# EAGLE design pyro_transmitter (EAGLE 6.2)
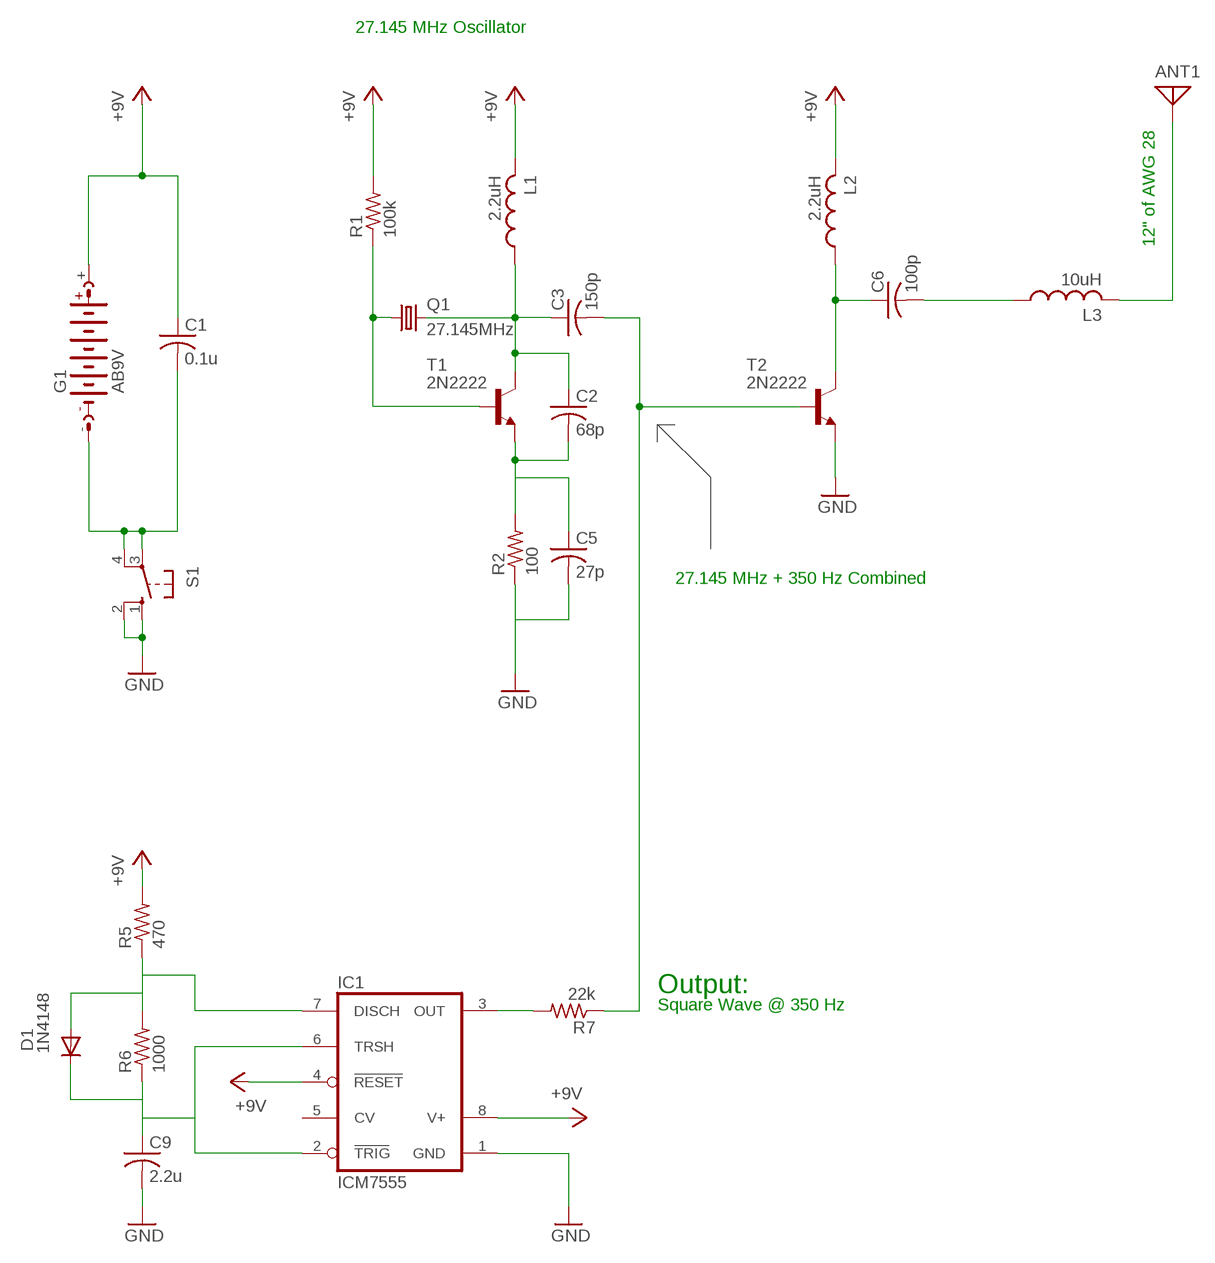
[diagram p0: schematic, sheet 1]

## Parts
ANT1  ANTENNA  [PAD-01]
C1  0.1u  C-US025-025X050  [C025-025X050]
C2  68p  C-US025-025X050  [C025-025X050]
C3  150p  C-US025-025X050  [C025-025X050]
C5  27p  C-US025-025X050  [C025-025X050]
C6  100p  C-US025-025X050  [C025-025X050]
C9  2.2u  C-US025-025X050  [C025-025X050]
D1  1N4148  1N4148DO35-7  [DO35-7]
G1  AB9V  [AB9V]
IC1  ICM7555  [DIL08]
L1  2.2uH  L-US0207/10  [0207/10]
L2  2.2uH  L-US0207/10  [0207/10]
L3  10uH  L-US0207/10  [0207/10]
Q1  27.145MHz  CRYSTALHC18U-V  [HC18U-V]
R1  100k  R-US_0207/10  [0207/10]
R2  100  R-US_0207/10  [0207/10]
R5  470  R-US_0207/10  [0207/10]
R6  1000  R-US_0207/10  [0207/10]
R7  22k  R-US_0207/10  [0207/10]
S1  10-XX  [B3F-10XX]
T1  2N2222  2N2222-NPN-TO92-EBC  [TO92-EBC]
T2  2N2222  2N2222-NPN-TO92-EBC  [TO92-EBC]

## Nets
+5V: C1.1 G1.+ IC1.4(RESET) IC1.8(V+) L1.2 L2.2 R1.2 R5.2 ; supply symbol labelled +9V
GND: C5.2 C9.2 IC1.1(GND) R2.1 S1.1(S) S1.2(S1) T2.E
N$1: C1.2 G1.- S1.3(P) S1.4(P1)
N$2: ANT1.1 L3.2
N$3: C2.1 C3.1 L1.1 Q1.2 T1.C
N$4: Q1.1 R1.1 T1.B
N$5: C2.2 C5.1 R2.2 T1.E
N$6: C3.2 R7.1 T2.B
N$8: C6.1 L2.1 T2.C
N$9: C6.2 L3.1
N$11: D1.A IC1.7(DISCH) R5.1 R6.2
N$12: C9.1 D1.C IC1.2(TRIG) IC1.6(TRSH) R6.1
N$13: IC1.3(OUT) R7.2
Unconnected: IC1.5(CV)

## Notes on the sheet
- 27.145 MHz Oscillator
- 12" of AWG 28
- 27.145 MHz + 350 Hz Combined
- Output:
- Square Wave @ 350 Hz

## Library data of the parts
ANT1 = discrete:ANTENNA: Antenna
C1-C3 C5 C6 C9 = resistor:C-US: CAPACITOR, American symbol
D1 = diode:1N4148: DIODE
G1 = battery:AB9V: 9-V BATTERY CLIP
IC1 = maxim:ICM7555: TIMER
L1-L3 = resistor:L-US: INDUCTOR, American symbol
Q1 = crystal:CRYSTAL: CRYSTAL
R1 R2 R5-R7 = resistor:R-US_: RESISTOR, American symbol
S1 = switch-omron:10-XX: OMRON SWITCH
T1 T2 = transistor-neu-to92:*-NPN-: NPN Transistror

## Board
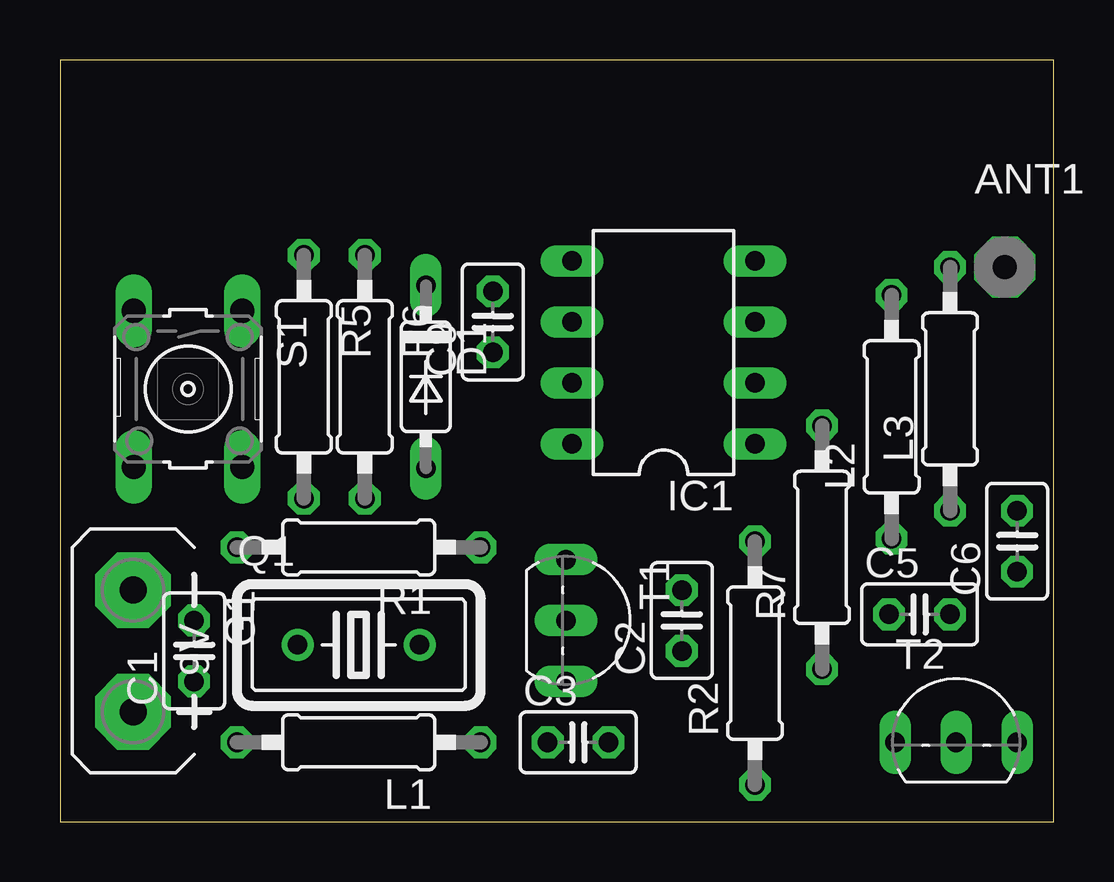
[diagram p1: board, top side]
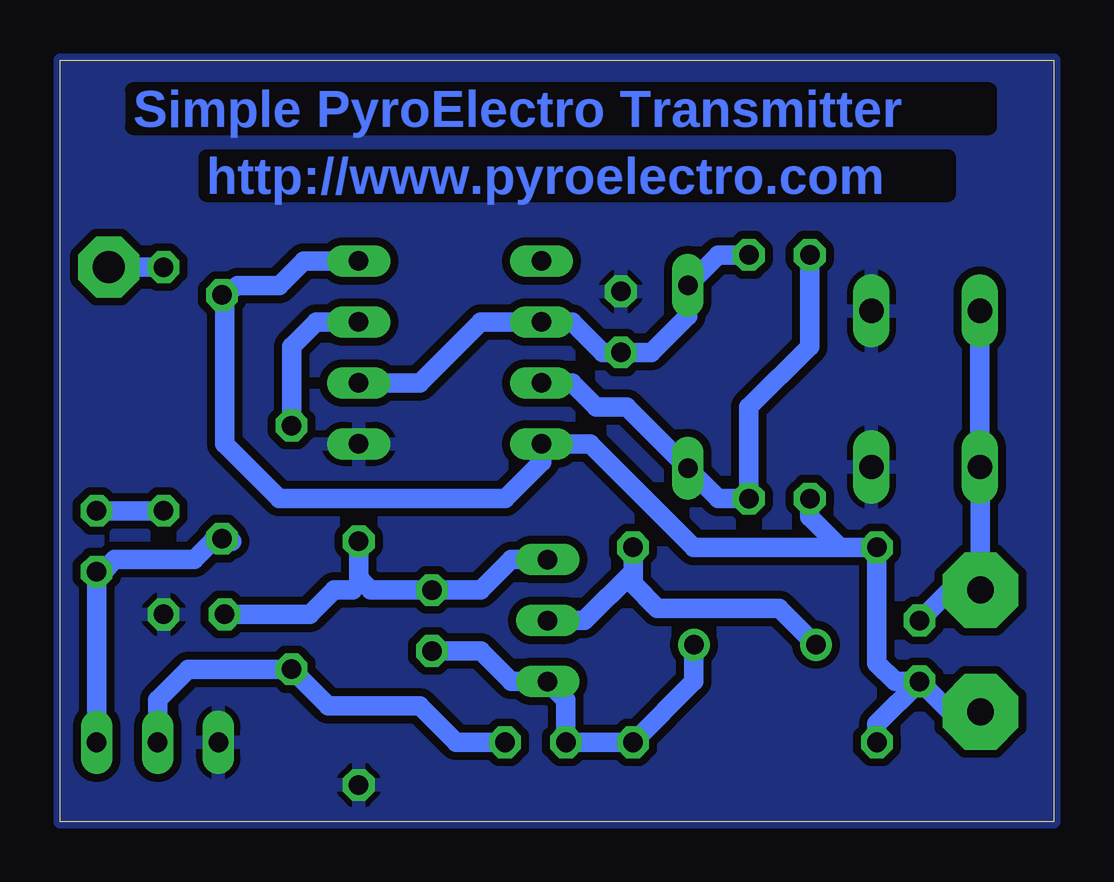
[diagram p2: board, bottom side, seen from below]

Size 41.4 x 31.75 mm. Coordinates in mm from the lower left corner, seen from the top.
Outline: 0,0 41.4,0 41.4,31.75 0,31.75 0,0
Copper layers (1*16): Top 0.035mm / dielectric 1.5mm / Bottom 0.035mm
Design rules: minimum track width 10mil, minimum drill 24mil, track to track 8mil, track to pad 8mil, pad to pad 8mil, via to via 8mil, smd to smd 8mil, copper to edge 0mil, drill to drill 8mil, minimum pad ring 10mil, minimum via ring 8mil, stop-mask expansion 4mil, vias tented up to drill 0mil, thermal gap 10mil

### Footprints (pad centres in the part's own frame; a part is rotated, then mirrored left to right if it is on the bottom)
PAD-01 = drill 1.321 pad 2.54 octagon: 1 0,0
C025-025X050 = drill 0.813 octagon: 1 -1.27,0; 2 1.27,0
DO35-7 = drill 0.813 long: A 3.81,0; C -3.81,0
AB9V = drill 1.118 pad 3.15 octagon: + 0,2.54; - 0,-2.54
DIL08 = drill 0.813 long: 1 -3.81,-3.81; 2 -1.27,-3.81; 3 1.27,-3.81; 4 3.81,-3.81; 5 3.81,3.81; 6 1.27,3.81; 7 -1.27,3.81; 8 -3.81,3.81
0207/10 = drill 0.813 octagon: 1 -5.08,0; 2 5.08,0
HC18U-V = drill 0.813: 1 -2.54,0; 2 2.54,0
B3F-10XX = drill 1.016 long: 1 -3.251,2.261; 2 3.251,2.261; 3 -3.251,-2.261; 4 3.251,-2.261
TO92-EBC = drill 0.813 long: B 0,-1.27; C 2.54,-1.27; E -2.54,-1.27

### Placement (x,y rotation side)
ANT1  39.37,23.11 0 top
C1  5.59,7.11 90 top
C2  25.91,8.38 90 top
C3  21.59,3.3 0 top
C5  35.81,8.64 0 top
C6  39.88,11.68 90 top
C9  18.03,20.83 90 top
D1  15.24,18.54 270 top
G1  3.05,7.11 180 top
IC1  25.15,19.56 90 top
L1  12.45,3.3 180 top
L2  34.65,16.87 90 top
L3  37.08,18.03 90 top
Q1  12.45,7.37 0 top
R1  12.45,11.43 180 top
R2  28.96,6.6 90 top
R5  10.16,18.54 270 top
R6  12.7,18.54 270 top
R7  31.75,11.43 90 top
S1  5.33,18.03 270 top
T1  22.35,8.38 270 top
T2  37.34,4.57 0 top

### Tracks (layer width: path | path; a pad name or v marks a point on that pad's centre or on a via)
+5V
  Bottom 0.813: G1.+ 4.32,4.57 C1.1 | L1.2 7.37,4.06 C1.1 | C1.1 6.6,5.84 7.37,6.6 R1.2 8.89,11.43 | 8.89,11.43 14.99,11.43 19.3,15.75 IC1.8 21.34,14.99 22.86,13.46 32.26,13.46 34.54,15.75 34.54,21.84 L2.2 33.99,22.35 32.26,22.35 31.24,23.37 IC1.4 | R5.2 10.16,12.7 8.89,11.43
GND
  pour Bottom (isolate 0.33): 0,0 0,31.75 41.4,31.75 41.4,0
N$1
  Bottom 0.813: C1.2 4.32,9.65 G1.- 3.05,14.76 S1.4 S1.3
N$2
  Bottom 0.813: L3.2 ANT1.1
N$3
  Bottom 0.813: Q1.2 14.99,5.84 L1.1 C3.1 20.32,5.08 T1.C 22.61,5.84 23.88,7.11 C2.1
N$4
  Bottom 0.813: Q1.1 11.43,8.89 16.51,8.89 17.53,9.91 17.53,10.41 | 17.53,10.41 R1.1 | T1.B 19.56,8.38 17.53,10.41
N$5
  Bottom 0.813: T1.E 22.61,10.92 23.88,9.65 C2.2 28.45,9.65 28.83,10.03 | 28.83,10.03 28.96,10.16 R2.2 | C5.1 30.99,8.64 29.97,9.65 29.21,9.65 28.83,10.03
N$6
  Bottom 0.813: C3.2 24.89,3.3 26.42,4.83 30.23,4.83 R7.1 36.07,6.35 37.34,5.08 T2.B
N$8
  Bottom 0.813: T2.C C6.1 39.62,10.41 39.12,10.92 35.81,10.92 35.05,11.68 34.25,11.68 L2.1
N$9
  Bottom 0.813: L3.1 C6.2
N$11
  Bottom 0.813: R5.1 10.16,19.81 12.7,17.27 R6.2 13.97,13.46 D1.A 17.78,17.27 19.05,17.27 20.07,18.29 IC1.7
N$12
  Bottom 0.813: R6.1 13.97,23.62 D1.C 15.24,21.08 16.76,19.56 C9.1 18.8,19.56 20.07,20.83 IC1.6 23.88,20.83 26.42,18.29 IC1.2
N$13
  Bottom 0.813: IC1.3 30.73,20.83 31.75,19.81 R7.2

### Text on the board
Bottom: Simple PyroElectro Transmitter | http://www.pyroelectro.com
